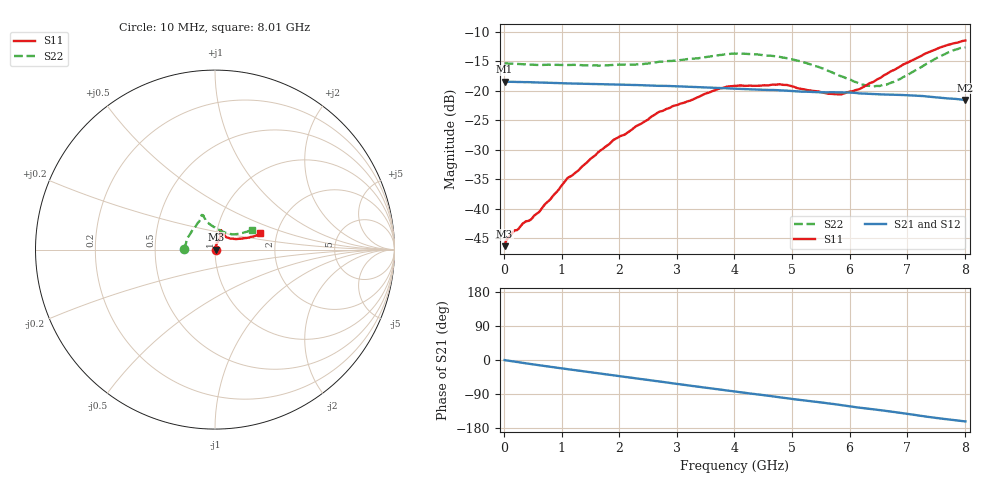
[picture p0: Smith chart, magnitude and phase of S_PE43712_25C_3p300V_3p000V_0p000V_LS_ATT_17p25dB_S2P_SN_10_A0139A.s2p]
! DEVICE ID: PE43712
! File Path: z:\PE43713\PE43713_CHAR_NOM_04292014\AMB\3p300\LS_ATT_17p25dB\PE43713_AMB_3p300V_3p000V_0p000V_LS_ATT_17p25dB_S2P_SN_10_A0139A.s2p
! Serial: 10
! Lot: A0139A
! Temp: 25C
! VDD: 3.300
! VSS: 0.000
! Control_Hi: 3.000
! Control_Lo: 0.000
! Attenuation Step: 17.25dB
! Port 1: RF1
! Port 2: RF2
! ThroughPath:1-2
! IDD: 0.0001467323
! ISS: -1.295e-007
#  Hz  S  RI  R  50
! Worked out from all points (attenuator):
!   801 points, 10 MHz to 8.01 GHz, reference 50 ohm
!   highest |S21| = -18.47 dB at 10 MHz (marker M1); lowest = -21.6 dB at 8.01 GHz (marker M2)
!   lowest |S11| = -46.3 dB at 10 MHz (marker M3), VSWR 1.01, Z = 50.5 + j0.0431 ohm
!   |S11| at or under -10 dB: start of sweep to end of sweep
!   |S22| runs from -19.3 to -12.6 dB; largest |S21 - S12| = 0.00043
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1e7  0.00481 0.000427  0.1193 -0.000638  0.1193 -0.000611  -0.1712 0.00116
1.6e8  0.0059 0.00243  0.1187 -0.00782  0.1187 -0.0078  -0.1689 0.0111
4.6e8  0.00599 0.00545  0.116 -0.0216  0.116 -0.0215  -0.1644 0.0268
6e8  0.0055 0.00753  0.1142 -0.0275  0.1142 -0.0275  -0.1617 0.0348
1.09e9  0.00472 0.0173  0.1055 -0.0468  0.1056 -0.0468  -0.1533 0.0615
1.35e9  0.00579 0.022  0.1001 -0.0559  0.1001 -0.056  -0.1472 0.0736
1.9e9  0.0116 0.0365  0.086 -0.0733  0.086 -0.0733  -0.1293 0.1035
2.35e9  0.0186 0.0481  0.0721 -0.0852  0.072 -0.0852  -0.1119 0.1241
2.68e9  0.0256 0.0607  0.061 -0.0916  0.061 -0.0916  -0.0984 0.1457
3.72e9  0.0322 0.0985  0.0228 -0.103  0.0227 -0.103  -0.0747 0.1852
4.01e9  0.0323 0.1052  0.0121 -0.1034  0.0121 -0.1034  -0.0743 0.1928
4.79e9  0.0331 0.1085  -0.015 -0.0997  -0.015 -0.0998  -0.0627 0.1829
5.35e9  0.0441 0.0896  -0.0321 -0.0923  -0.0321 -0.0923  -0.0487 0.1584
5.64e9  0.0542 0.0771  -0.04 -0.0883  -0.04 -0.0883  -0.0313 0.1434
5.87e9  0.0639 0.0684  -0.0472 -0.0844  -0.0471 -0.0845  -0.0136 0.1311
6.17e9  0.0824 0.0622  -0.0555 -0.0771  -0.0553 -0.0771  0.0144 0.1136
6.38e9  0.1 0.0612  -0.0596 -0.0722  -0.0595 -0.0722  0.0372 0.1023
6.68e9  0.1298 0.0597  -0.0659 -0.0651  -0.0658 -0.0651  0.0722 0.0894
6.99e9  0.1595 0.0631  -0.0722 -0.0567  -0.072 -0.0566  0.1037 0.0854
7.37e9  0.1996 0.0707  -0.0774 -0.0442  -0.0773 -0.0442  0.1467 0.0912
7.72e9  0.2322 0.0793  -0.0791 -0.0337  -0.0791 -0.0337  0.1854 0.1028
8.01e9  0.2509 0.0898  -0.0795 -0.0256  -0.0794 -0.0257  0.2056 0.1103
